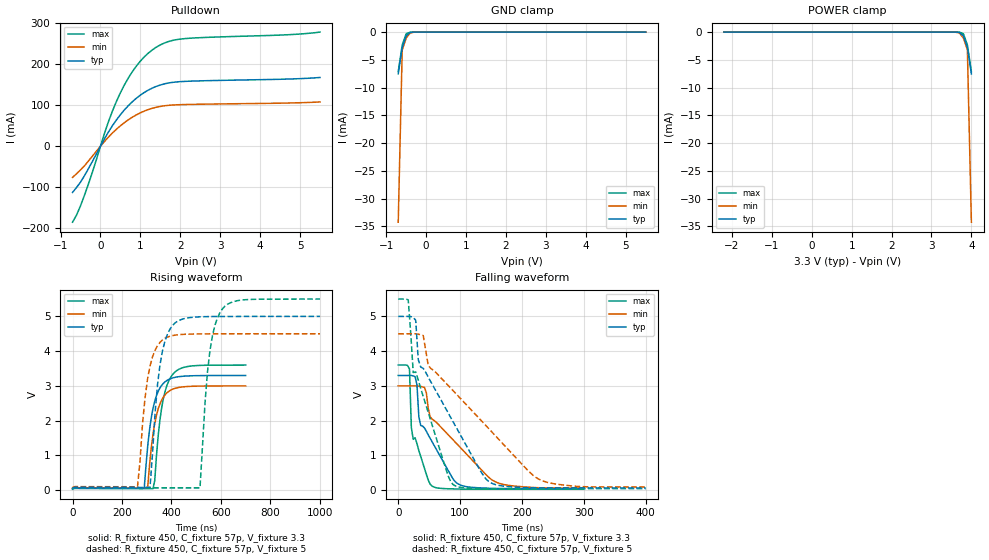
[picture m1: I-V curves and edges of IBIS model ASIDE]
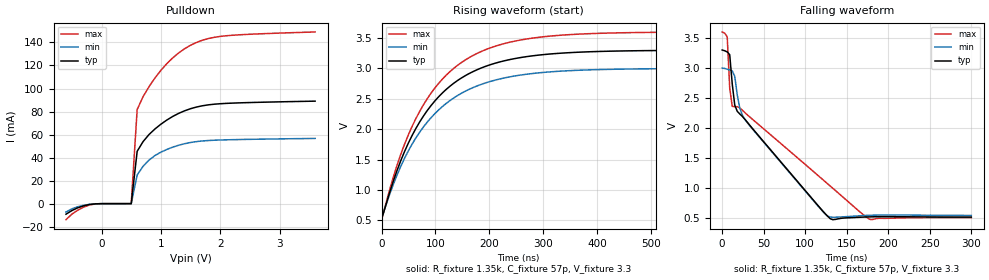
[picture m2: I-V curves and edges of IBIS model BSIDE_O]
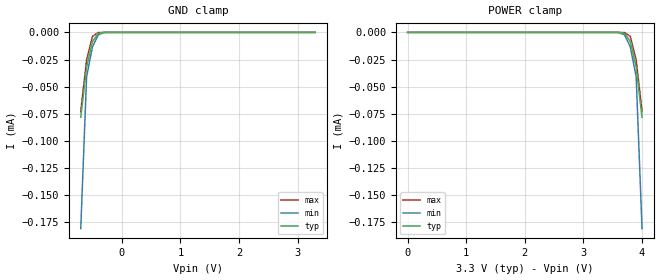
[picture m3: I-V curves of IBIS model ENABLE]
[IBIS Ver]   3.2
[Comment Char]   |_char
| VDD nom: 3.3v, min: 3v, max:3.6v
[File name]   pca9507_a_3_3.ibs
[File Rev]   1
[Date]   Sep 19, 2008 11:25:36 AM
[Source]
Generated using IBISToolkit at NXP Tempe by Seshadri Venkataramanan
[Notes]
[Disclaimer]
(C) Copyright 2007 NXP Semiconductors
All rights reserved
NXP Semiconductors (NXP) does not warrant that this model and any other
accompanying information (Model) accurately or fully represents the
operating characteristics and specifications of the semiconductor
products to which the Model relates.  Moreover, the Model is furnished
on an "as is" and with "all faults" basis, and without support or
warranty of any kind.  NXP disclaims all warranties, whether expressed
or implied or statutory, including without limitation all implied
warranties of non-infringement, merchantability and fitness for any
purpose, and those arising from a course of dealing or usage of trade.
NXP does not convey any license under its or any third party's patents,
copyrights or other intellectual property or proprietary rights.
You and your company assume any and all risks and liability arising out
of the application or use of the Model.
In no event shall NXP be liable for any direct, indirect, special,
consequential or incidental damages, however caused, whether in
warranty, contract or tort (including negligence), strict liability or
other legal theory, including, without limitation, for lost profits,
business interruption, or corruption or loss of data or information,
arising out of or in connection with the use of or the inability to use
the Model, even if NXP has been advised of the possibility of such
damages.
NXP provides the Model as a courtesy to our customers. You and your
company shall not distribute, convey, sell, or give the Model to anyone
else without receiving prior written permission from NXP.
NXP reserves the right to make changes without notice to the Model to
improve reliability, function, or design.
Please be aware that your receipt and subsequent use of the Model shall
serve as acceptance of these terms and conditions.  If you do not
accept these terms, return or destroy the Model immediately.
[Copyright]
2008
| SO8
[Component]   PCA9507D
Si_location Pin
Timing_location Pin
[Manufacturer]   NXP
[Package]
R_pkg   4.81E-02   4.14E-02   5.47E-02
L_pkg   1.88n   1.54n   2.21n
C_pkg   4.49E-13   4.17E-13   4.81E-13
[Pin] signal_name   model_name   R_pin   L_pin   C_pin
1   VCCA   POWER   5.47E-02  2.21E-09  4.81E-13
2   SCLA   ASIDE   4.14E-02  1.54E-09  4.20E-13
3   SDAA   ASIDE   4.14E-02  1.55E-09  4.20E-13
4   GND   GND   5.47E-02  2.21E-09  4.80E-13
5   EN   ENABLE   5.47E-02  2.21E-09  4.78E-13
6   SDAB   BSIDE_I/O   4.14E-02  1.55E-09  4.17E-13
7   SCLB   BSIDE_I/O   4.14E-02  1.54E-09  4.17E-13
8   VCCB   POWER   5.47E-02  2.21E-09  4.79E-13
| TSSOP8
[Component]   PCA9507AD
Si_location Pin
Timing_location Pin
[Manufacturer]   NXP
[Package]
R_pkg   33.7m   30.1m   37.3m
L_pkg   1.74n   1.67n   1.81n
C_pkg   0.428p   0.422p   0.434p
[Pin] signal_name   model_name   R_pin   L_pin   C_pin
1   VCCA   POWER   37.3m   1.81nH   0.428pF
2   SCLA   ASIDE   30.1m   1.67nH   0.422pF
3   SDAA   ASIDE   30.1m   1.67nH   0.428pF
4   GND   GND   37.3m   1.81nH   0.434pF
5   EN   ENABLE   37.3m   1.81nH   0.428pF
6   SDAB   BSIDE_I/O   30.1m   1.67nH   0.422pF
7   SCLB   BSIDE_I/O   30.1m   1.67nH   0.428pF
8   VCCB   POWER   37.3m   1.81nH   0.434pF
[Model Selector]   BSIDE_I/O
BSIDE_I   Bside as Input
BSIDE_O   Bside as Output
| Models and submodels in the file (4): ASIDE (I/O_open_drain), BSIDE_O (Open_drain), ENABLE (Input), BSIDE_I (Input)
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[Model]   ASIDE
Model_type I/O_open_drain
Vinh=2.31
Vinl=0.99
Vref=3.3
Vmeas=1.65
Rref=450
Cref=57p
C_comp   5.2p   5p   5.4p
[Temperature Range] 27   85   -40
[Voltage Range]   3.3   3   3.6
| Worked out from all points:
|   slope of the pulldown table from 0 to 0.495 V, typ, clamps not added: 6.49 ohm
|   GND clamp passes 1 mA (typ) near -0.52 V on its own axis
|   falling waveform, R_fixture 450, C_fixture 57p, V_fixture 3.3: 20-80 % time 45.1ns typ, 83ns min, 21.1ns max; typ from 3.3 V to 0.04 V
|   falling waveform, R_fixture 450, C_fixture 57p, V_fixture 5: 20-80 % time 85.9ns typ, 140ns min, 47.2ns max; typ from 5 V to 0.061 V
|   rising waveform, R_fixture 450, C_fixture 57p, V_fixture 3.3: 20-80 % time 39.4ns typ, 39.5ns min, 39ns max; typ from 0.04 V to 3.3 V
|   rising waveform, R_fixture 450, C_fixture 57p, V_fixture 5: 20-80 % time 40.5ns typ, 40.9ns min, 40.5ns max; typ from 0.061 V to 5 V
[Pulldown]
-700mV    -112.8mA   -76.07mA   -185.2mA
-600mV    -100.6mA   -67.26mA   -168mA
-400mV    -71.71mA   -47.72mA   -119.3mA
-200mV    -36.74mA   -23.97mA   -62.63mA
200mV     34.61mA    22.2mA     59.69mA
500mV     76.81mA    49.77mA    130.3mA
700mV     99.01mA    64.46mA    166.5mA
900mV     117mA      76.37mA    195.3mA
1.3V      141.7mA    92.44mA    234.8mA
1.7V      153.9mA    99.55mA    254.9mA
2.1V      157.9mA    101.5mA    262.1mA
5.5V      167.4mA    107.8mA    278.1mA
[GND Clamp]
-700mV    -7.515mA   -34.24mA   -7.132mA
-600mV    -2.755mA   -3.204mA   -2.308mA
-500mV    -688.7uA   -1.069mA   -295.9uA
-400mV    -56.82uA   -166.8uA   -8.054uA
-200mV    -26.66nA   -203.8nA   -742.7pA
5.5V      383.1pA    684.5pA    354.1pA
[POWER Clamp]
-2.2V     383.1pA    684.5pA    354.1pA
3.5V      -26.66nA   -203.8nA   -742.7pA
3.7V      -56.82uA   -166.8uA   -8.054uA
3.8V      -688.7uA   -1.069mA   -295.9uA
3.9V      -2.755mA   -3.204mA   -2.308mA
4V        -7.515mA   -34.24mA   -7.132mA
[Falling Waveform]
R_fixture=450
C_fixture=57p
V_fixture=3.3
V_fixture_min=3
V_fixture_max=3.6
0s        3.3V       3V         3.6V
18.18ns   3.3V       3V         3.485V
21.21ns   3.299V     3V         1.795V
24.24ns   3.286V     3V         1.46V
30.3ns    3.026V     3V         1.336V
36.36ns   1.858V     2.983V     966.9mV
54.55ns   1.396V     2.046V     117.3mV
103ns     128.3mV    1.175V     27.45mV
163.6ns   43.11mV    192.3mV    25.46mV
300ns     40.19mV    57.61mV    25.38mV
[Falling Waveform]
R_fixture=450
C_fixture=57p
V_fixture=5
V_fixture_min=4.5
V_fixture_max=5.5
0s        5V         4.5V       5.5V
16.16ns   5V         4.5V       5.477V
24.24ns   4.976V     4.5V       3.385V
28.28ns   4.886V     4.499V     3.401V
36.36ns   3.543V     4.471V     2.919V
48.48ns   3.251V     3.591V     2.235V
88.89ns   1.96V      2.859V     155.3mV
153.5ns   178.3mV    1.631V     39.97mV
234.3ns   62.63mV    258.8mV    39.21mV
400ns     61.43mV    86.93mV    39.15mV
[Rising Waveform]
R_fixture=450
C_fixture=57p
V_fixture=3.3
V_fixture_min=3
V_fixture_max=3.6
0s        40.1mV     56.98mV    25.36mV
289.9ns   57.19mV    60.7mV     40.48mV
304ns     1.28V      101.1mV    40.27mV
325.3ns   2.35V      1.609V     40.06mV
332.3ns   2.559V     1.918V     274.5mV
346.5ns   2.845V     2.343V     1.581V
360.6ns   3.016V     2.595V     2.382V
403ns     3.224V     2.898V     3.312V
473.7ns   3.287V     2.984V     3.566V
700ns     3.298V     2.999V     3.598V
[Rising Waveform]
R_fixture=450
C_fixture=57p
V_fixture=5
V_fixture_min=4.5
V_fixture_max=5.5
0s        61.32mV    86.34mV    39.12mV
262.6ns   74.93mV    94.31mV    62.76mV
292.9ns   74.46mV    2.642V     62.1mV
313.1ns   74.36mV    3.569V     61.88mV
343.4ns   3.029V     4.156V     61.72mV
373.7ns   4.292V     4.37V      61.64mV
515.2ns   4.987V     4.495V     61.51mV
545.5ns   4.993V     4.496V     3.404V
596ns     4.997V     4.498V     5.111V
1us       4.999V     4.499V     5.498V
[Ramp]
R_load=450
dV/dt_r   1.794E+0/1.740E-9   2.253E-3/3.574E-10   8.971E-3/3.418E-10
dV/dt_f   1.956E+0/4.456E-8   1.942E+0/9.511E-8   1.966E+0/1.632E-8
|[End   ASIDE
[Model]   BSIDE_O
Model_type Open_drain
Vref=3.3
Vmeas=1.65
Rref=1.35k
Cref=57p
C_comp   4.8p   4.6p   5p
[Temperature Range] 27   85   -40
[Voltage Range]   3.3   3   3.6
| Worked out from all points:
|   slope of the pulldown table from 0 to 0.495 V, typ, clamps not added: 32 kohm
|   falling waveform, R_fixture 1.35k, C_fixture 57p, V_fixture 3.3: 20-80 % time 80.9ns typ, 76.1ns min, 114ns max; typ from 3.3 V to 0.519 V
|   rising waveform, R_fixture 1.35k, C_fixture 57p, V_fixture 3.3: 20-80 % time 113ns typ, 114ns min, 113ns max; typ from 0.523 V to 3.3 V
[Pulldown]
-600mV    -9.162mA   -7.275mA   -13.93mA
-400mV    -3.57mA    -2.706mA   -5.622mA
-200mV    -721.5uA   -570.6uA   -1.102mA
500mV     6.358uA    5.585uA    4.121uA
600mV     45.46mA    24.83mA    81.73mA
700mV     53.91mA    32.44mA    92.96mA
900mV     64.85mA    41.77mA    109.2mA
1.1V      72.61mA    47.07mA    121.6mA
1.3V      78.41mA    50.72mA    130.9mA
1.6V      83.9mA     53.89mA    140mA
1.9V      86.37mA    55.08mA    144.5mA
3.6V      89.02mA    56.64mA    149.1mA
[Falling Waveform]
R_fixture=1.35k
C_fixture=57p
V_fixture=3.3
V_fixture_min=3
V_fixture_max=3.6
0s        3.3V       3V         3.6V
6.061ns   3.268V     2.98V      3.52V
9.091ns   3.222V     2.967V     2.664V
12.12ns   2.736V     2.954V     2.363V
15.15ns   2.383V     2.861V     2.356V
21.21ns   2.235V     2.332V     2.336V
27.27ns   2.148V     2.148V     2.259V
130.3ns   490.4mV    519.5mV    1.033V
178.8ns   522.4mV    549.1mV    476.2mV
300ns     518.8mV    546mV      509.9mV
[Rising Waveform]
R_fixture=1.35k
C_fixture=57p
V_fixture=3.3
V_fixture_min=3
V_fixture_max=3.6
0s        522.6mV    549.6mV    511.8mV
21.21ns   1.132V     1.08V      1.197V
35.35ns   1.477V     1.384V     1.581V
56.57ns   1.895V     1.754V     2.045V
77.78ns   2.217V     2.038V     2.402V
120.2ns   2.656V     2.425V     2.89V
176.8ns   2.975V     2.709V     3.243V
240.4ns   3.149V     2.864V     3.434V
332.3ns   3.249V     2.954V     3.545V
700ns     3.298V     2.999V     3.598V
[Ramp]
R_load=1350
dV/dt_r   1.666E+0/7.705E-9   1.649E+0/7.656E-9   1.673E+0/7.525E-9
dV/dt_f   1.669E+0/7.512E-8   1.652E+0/8.638E-8   1.674E+0/8.557E-8
|[End   BSIDE_O
[Model]   ENABLE
Model_type Input
Vinh=2.31
Vinl=0.99
C_comp   1.7p   1.5p   1.9p
[Temperature Range] 27   85   -40
[Voltage Range]   3.3   3   3.6
[GND Clamp]
-700mV    -78.2uA    -180.8uA   -72.93uA
-600mV    -31.83uA   -40.84uA   -25.27uA
-500mV    -8.452uA   -13.3uA    -3.68uA
-400mV    -758.4nA   -2.213uA   -96.83nA
-300mV    -18.6nA    -106.4nA   -805pA
-200mV    -273.4pA   -2.436nA   -5.553pA
3.3V      6.665pA    8.025pA    6.6pA
[POWER Clamp]
0V        6.665pA    8.025pA    6.6pA
3.5V      -273.4pA   -2.436nA   -5.553pA
3.6V      -18.6nA    -106.4nA   -805pA
3.7V      -758.4nA   -2.213uA   -96.83nA
3.8V      -8.452uA   -13.3uA    -3.68uA
3.9V      -31.83uA   -40.84uA   -25.27uA
4V        -78.2uA    -180.8uA   -72.93uA
